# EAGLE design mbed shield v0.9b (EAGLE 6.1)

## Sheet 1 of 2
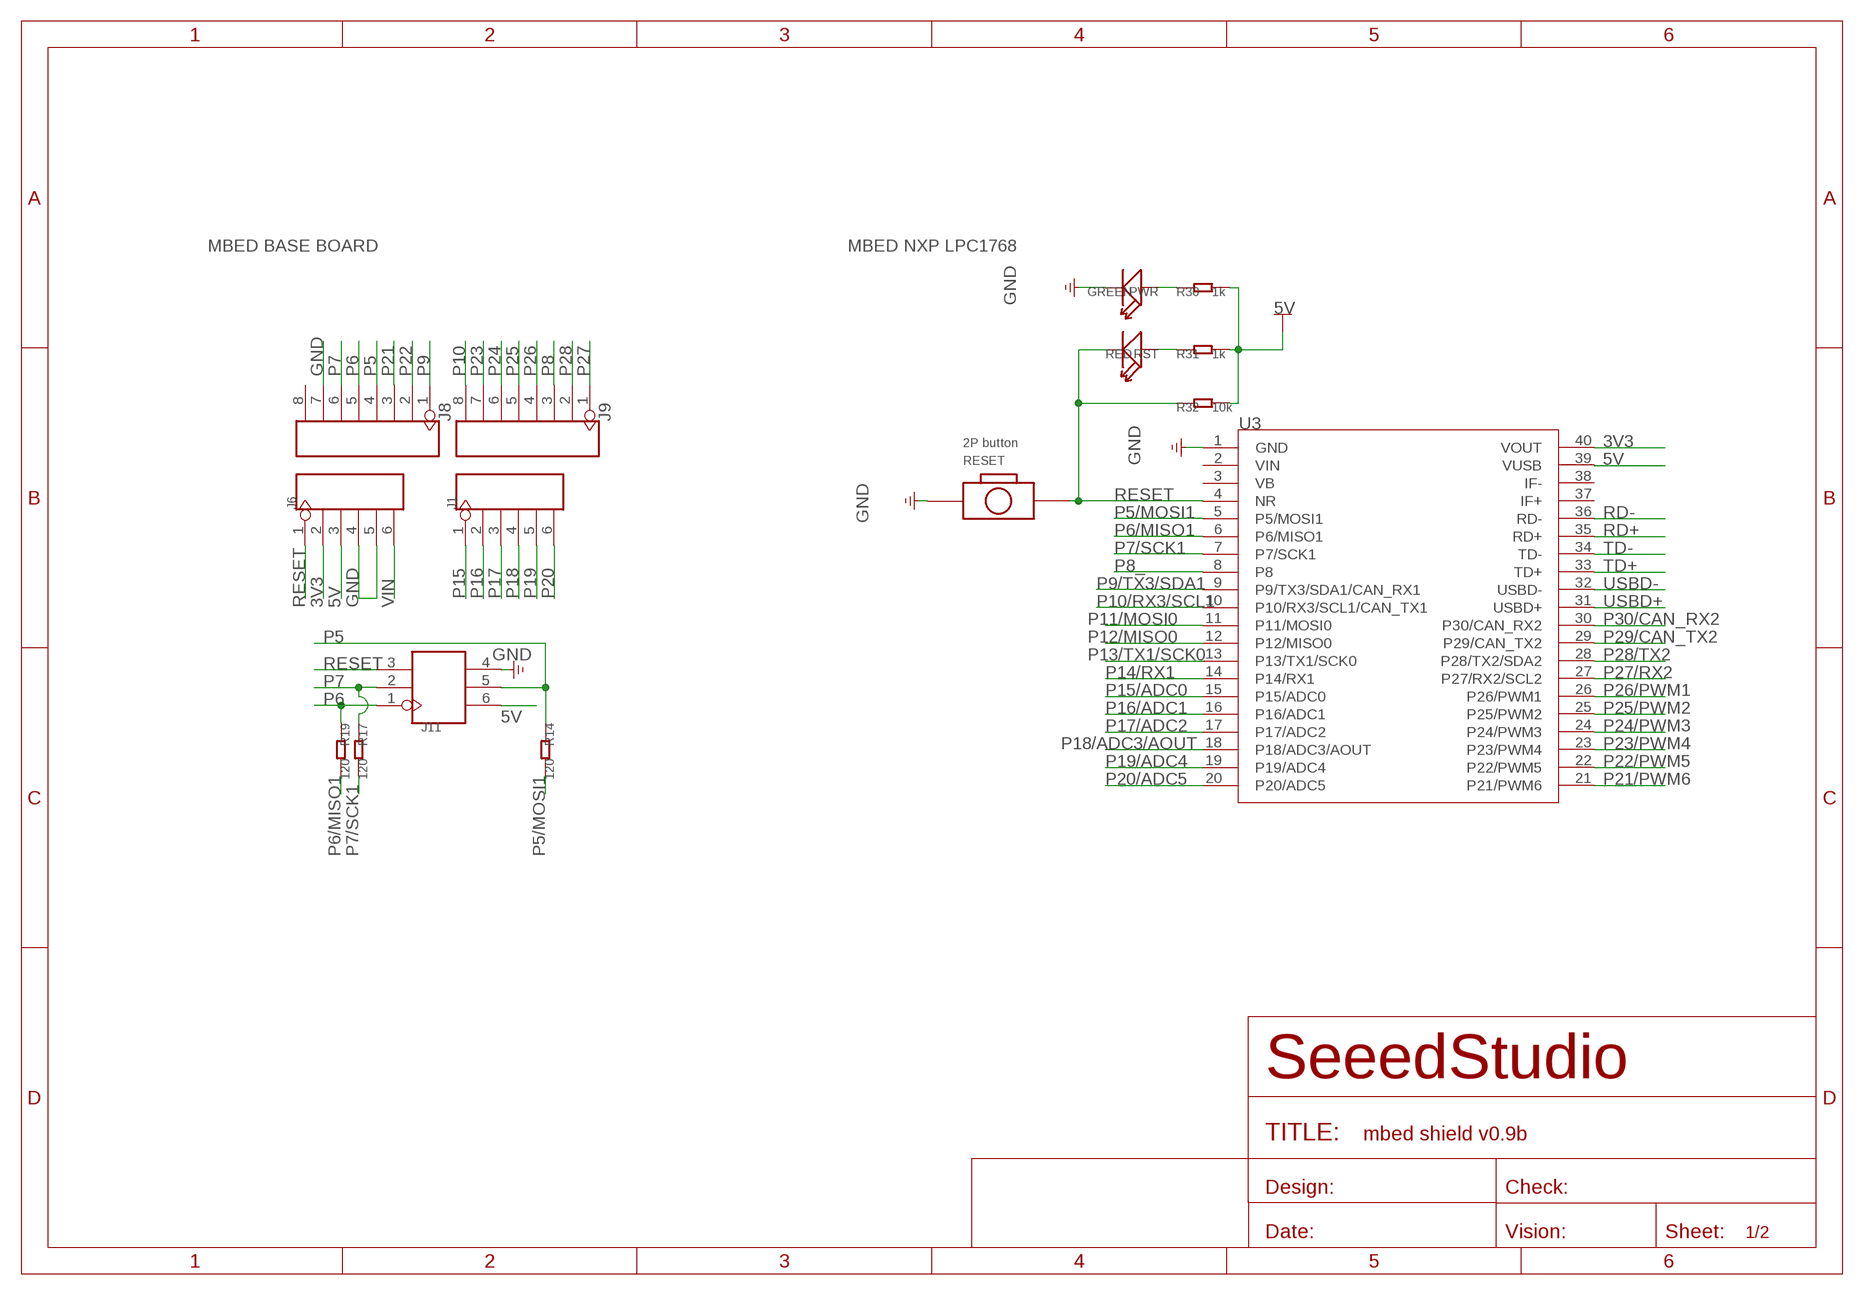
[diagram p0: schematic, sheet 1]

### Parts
J1  HEADER-6P-SMD  [6P-2.54-SMD]
J6  HEADER-6P-SMD  [6P-2.54-SMD]
J8  HEADER-8P-2.54-SMD  [8P-2.54-SMD]
J9  HEADER-8P-2.54-SMD  [8P-2.54-SMD]
J11  HEADER-2X3P-2.54  [2X3P-2.54]
PWR  GREEN  LED'0603'  [LED-0603]
R14  120  R-0603  [0603]
R17  120  R-0603  [0603]
R19  120  R-0603  [0603]
R30  1k  R-0603  [0603]
R31  1k  R-0603  [0603]
R32  10k  R-0603  [0603]
RESET  2P button  BOTTON-2P-90  [2P-7.62X3.56-90D]
RST  RED  LED'0603'  [LED-0603]
U3  MBED-LPC1768-SMD  [40P-SMD-2.54-53.34X36.67]

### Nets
3V3: J6.2 U3.40(VOUT) ; also sheet 2
5V: J6.3 J11.6 R30.2 R31.2 R32.2 U3.39(VUSB) ; also sheet 2
GND: J6.4 J6.5 J8.7 J11.4 PWR.- RESET.P$1 U3.1(GND) ; also sheet 2
N$2: R31.1 RST.+
N$3: PWR.+ R30.1
P5: J8.4 J11.5 R14.1
P5/MOSI1: R14.2 U3.5(P5/MOSI1)
P6: J8.5 J11.1 R19.1
P6/MISO1: R19.2 U3.6(P6/MISO1)
P7: J8.6 J11.2 R17.1
P7/SCK1: R17.2 U3.7(P7/SCK1)
P8: J9.3 ; also sheet 2
P8_: U3.8 ; also sheet 2
P9: J8.1 ; also sheet 2
P9/TX3/SDA1: U3.9(P9/TX3/SDA1/CAN_RX1) ; also sheet 2
P10: J9.8 ; also sheet 2
P10/RX3/SCL1: U3.10(P10/RX3/SCL1/CAN_TX1) ; also sheet 2
P11/MOSI0: U3.11(P11/MOSI0) ; also sheet 2
P12/MISO0: U3.12(P12/MISO0) ; also sheet 2
P13/TX1/SCK0: U3.13(P13/TX1/SCK0) ; also sheet 2
P14/RX1: U3.14(P14/RX1) ; also sheet 2
P15: J1.1 ; also sheet 2
P15/ADC0: U3.15(P15/ADC0) ; also sheet 2
P16: J1.2 ; also sheet 2
P16/ADC1: U3.16(P16/ADC1) ; also sheet 2
P17: J1.3 ; also sheet 2
P17/ADC2: U3.17(P17/ADC2) ; also sheet 2
P18: J1.4 ; also sheet 2
P18/ADC3/AOUT: U3.18(P18/ADC3/AOUT) ; also sheet 2
P19: J1.5 ; also sheet 2
P19/ADC4: U3.19(P19/ADC4) ; also sheet 2
P20: J1.6 ; also sheet 2
P20/ADC5: U3.20(P20/ADC5) ; also sheet 2
P21: J8.3 ; also sheet 2
P21/PWM6: U3.21(P21/PWM6) ; also sheet 2
P22: J8.2 ; also sheet 2
P22/PWM5: U3.22(P22/PWM5) ; also sheet 2
P23: J9.7 ; also sheet 2
P23/PWM4: U3.23(P23/PWM4) ; also sheet 2
P24: J9.6 ; also sheet 2
P24/PWM3: U3.24(P24/PWM3) ; also sheet 2
P25: J9.5 ; also sheet 2
P25/PWM2: U3.25(P25/PWM2) ; also sheet 2
P26: J9.4 ; also sheet 2
P26/PWM1: U3.26(P26/PWM1) ; also sheet 2
P27: J9.1 ; also sheet 2
P27/RX2: U3.27(P27/RX2/SCL2) ; also sheet 2
P28: J9.2 ; also sheet 2
P28/TX2: U3.28(P28/TX2/SDA2) ; also sheet 2
P29/CAN_TX2: U3.29(P29/CAN_TX2) ; also sheet 2
P30/CAN_RX2: U3.30(P30/CAN_RX2) ; also sheet 2
RD+: U3.35(RD+) ; also sheet 2
RD-: U3.36(RD-) ; also sheet 2
RESET: J6.1 J11.3 R32.1 RESET.P$2 RST.- U3.4(NR)
TD+: U3.33(TD+) ; also sheet 2
TD-: U3.34(TD-) ; also sheet 2
USBD+: U3.31(USBD+) ; also sheet 2
USBD-: U3.32(USBD-) ; also sheet 2
VIN: J6.6
Unconnected: J8.8 U3.2(VIN) U3.3(VB) U3.37(IF+) U3.38(IF-)

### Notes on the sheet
- MBED BASE BOARD | MBED NXP LPC1768

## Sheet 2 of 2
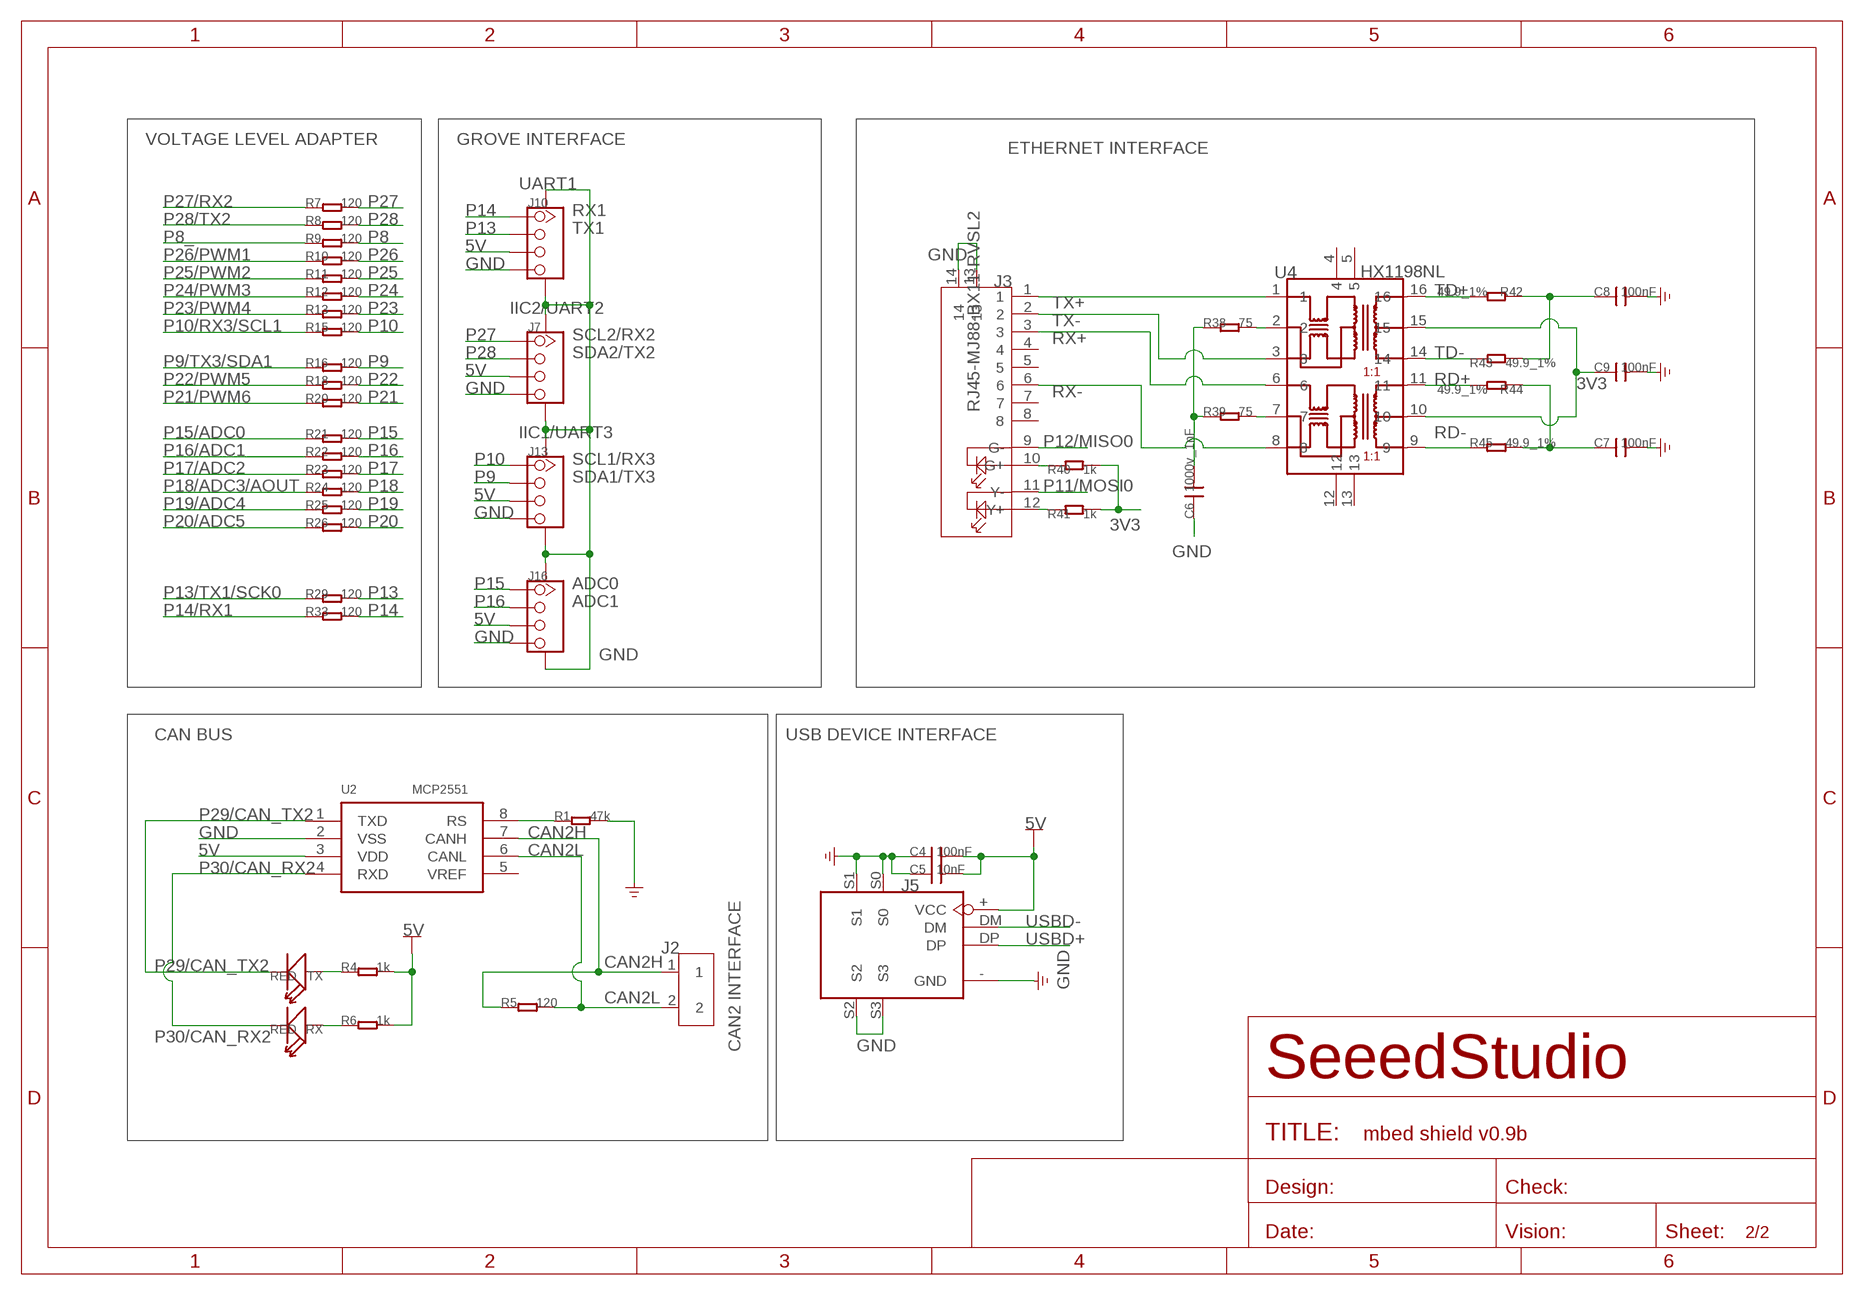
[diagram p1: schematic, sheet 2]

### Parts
C4  100nF  C-0603  [0603]
C5  10nF  C-0603  [0603]
C6  1000v_1nF  C  [C1206]
C7  100nF  C-0603  [0603]
C8  100nF  C-0603  [0603]
C9  100nF  C-0603  [0603]
J2  SCREW-TERMINAL-2P'3.5'  [2P-3.5]
J3  RJ45-MJ88-BX11-RVSL2  [RJ45-MJ88-BX11-RVSL2]
J5  USB-FEMALE-13.2X14.5  [FEMALE-14.5X13.2]
J7  TWIG-4P-2.0-SMD-FEMALE-REINFORCE'DD'  [4P-SMD-2.0]
J10  TWIG-4P-2.0-SMD-FEMALE-REINFORCE'DD'  [4P-SMD-2.0]
J13  TWIG-4P-2.0-SMD-FEMALE-REINFORCE'DD'  [4P-SMD-2.0]
J16  TWIG-4P-2.0-SMD-FEMALE-REINFORCE'DD'  [4P-SMD-2.0]
R1  47k  R-0603  [0603]
R4  1k  R-0603  [0603]
R5  120  R-0805  [0805]
R6  1k  R-0603  [0603]
R7  120  R-0603  [0603]
R8  120  R-0603  [0603]
R9  120  R-0603  [0603]
R10  120  R-0603  [0603]
R11  120  R-0603  [0603]
R12  120  R-0603  [0603]
R13  120  R-0603  [0603]
R15  120  R-0603  [0603]
R16  120  R-0603  [0603]
R18  120  R-0603  [0603]
R20  120  R-0603  [0603]
R21  120  R-0603  [0603]
R22  120  R-0603  [0603]
R23  120  R-0603  [0603]
R24  120  R-0603  [0603]
R25  120  R-0603  [0603]
R26  120  R-0603  [0603]
R29  120  R-0603  [0603]
R33  120  R-0603  [0603]
R38  75  R-0603  [0603]
R39  75  R-0603  [0603]
R40  1k  R-0603  [0603]
R41  1k  R-0603  [0603]
R42  49.9_1%  R-0603  [0603]
R43  49.9_1%  R-0603  [0603]
R44  49.9_1%  R-0603  [0603]
R45  49.9_1%  R-0603  [0603]
RX  RED  LED'0603'  [LED-0603]
TX  RED  LED'0603'  [LED-0603]
U2  MCP2551  [SO08]
U4  HX1198NL  [SOIC16-9.53]

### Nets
3V3: C9.1 R40.2 R41.2 U4.10 U4.15 ; also sheet 1
5V: C4.2 C5.2 J5.+(VCC) J7.3 J10.3 J13.3 J16.3 R4.2 R6.2 U2.3(VDD) ; also sheet 1
CAN2H: J2.1 R5.1 U2.7(CANH)
CAN2L: J2.2 R5.2 U2.6(CANL)
GND: C4.1 C5.1 C6.1 C7.2 C8.2 C9.2 J3.13 J3.14 J5.-(GND) J5.S0 J5.S1 J5.S2 J5.S3 J7.4 J7.SS1 J7.SS2 J10.4 J10.SS1 J10.SS2 J13.4 J13.SS1 J13.SS2 J16.4 J16.SS1 J16.SS2 R1.2 U2.2(VSS) ; also sheet 1
N$1: R39.2 U4.7
N$4: R38.2 U4.2
N$5: C6.2 R38.1 R39.1
N$6: C7.1 R44.1 R45.2
N$7: C8.1 R42.1 R43.2
N$11: J3.12(Y+) R41.1
N$12: J3.10(G+) R40.1
N$20: R1.1 U2.8(RS)
N$46: R4.1 TX.+
N$47: R6.1 RX.+
P8: R9.2 ; also sheet 1
P8_: R9.1 ; also sheet 1
P9: J13.2 R16.2 ; also sheet 1
P9/TX3/SDA1: R16.1 ; also sheet 1
P10: J13.1 R15.2 ; also sheet 1
P10/RX3/SCL1: R15.1 ; also sheet 1
P11/MOSI0: J3.11(Y-) ; also sheet 1
P12/MISO0: J3.9(G-) ; also sheet 1
P13: J10.2 R29.2
P13/TX1/SCK0: R29.1 ; also sheet 1
P14: J10.1 R33.2
P14/RX1: R33.1 ; also sheet 1
P15: J16.1 R21.2 ; also sheet 1
P15/ADC0: R21.1 ; also sheet 1
P16: J16.2 R22.2 ; also sheet 1
P16/ADC1: R22.1 ; also sheet 1
P17: R23.2 ; also sheet 1
P17/ADC2: R23.1 ; also sheet 1
P18: R24.2 ; also sheet 1
P18/ADC3/AOUT: R24.1 ; also sheet 1
P19: R25.2 ; also sheet 1
P19/ADC4: R25.1 ; also sheet 1
P20: R26.2 ; also sheet 1
P20/ADC5: R26.1 ; also sheet 1
P21: R20.2 ; also sheet 1
P21/PWM6: R20.1 ; also sheet 1
P22: R18.2 ; also sheet 1
P22/PWM5: R18.1 ; also sheet 1
P23: R13.2 ; also sheet 1
P23/PWM4: R13.1 ; also sheet 1
P24: R12.2 ; also sheet 1
P24/PWM3: R12.1 ; also sheet 1
P25: R11.2 ; also sheet 1
P25/PWM2: R11.1 ; also sheet 1
P26: R10.2 ; also sheet 1
P26/PWM1: R10.1 ; also sheet 1
P27: J7.1 R7.2 ; also sheet 1
P27/RX2: R7.1 ; also sheet 1
P28: J7.2 R8.2 ; also sheet 1
P28/TX2: R8.1 ; also sheet 1
P29/CAN_TX2: TX.- U2.1(TXD) ; also sheet 1
P30/CAN_RX2: RX.- U2.4(RXD) ; also sheet 1
RD+: R44.2 U4.11 ; also sheet 1
RD-: R45.1 U4.9 ; also sheet 1
RX+: J3.3 U4.6
RX-: J3.6 U4.8
TD+: R42.2 U4.16 ; also sheet 1
TD-: R43.1 U4.14 ; also sheet 1
TX+: J3.1 U4.1
TX-: J3.2 U4.3
USBD+: J5.DP ; also sheet 1
USBD-: J5.DM ; also sheet 1
Unconnected: J3.4 J3.5 J3.7 J3.8 U2.5(VREF) U4.4 U4.5 U4.12 U4.13

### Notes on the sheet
- VOLTAGE LEVEL ADAPTER | GROVE INTERFACE
- ETHERNET INTERFACE
- UART1
- RX1
- TX1
- IIC2/UART2
- SCL2/RX2
- SDA2/TX2
- IIC1/UART3
- SCL1/RX3
- SDA1/TX3
- ADC0
- ADC1
- CAN BUS | USB DEVICE INTERFACE
- CAN2 INTERFACE

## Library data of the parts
C4-C9 = Discrete:C*: Ceramic Capacitors
J1 J6 = Connector:HEADER-6P
J2 = Connector:SCREW-TERMINAL-2P
J3 = Connector:RJ45-MJ88-BX11-RVSL2: Modular Jack 8P8C,R/A,With LED
J5 = Connector:USB-FEMALE
J7 J10 J13 J16 = Connector:TWIG-4P-2.0-SMD-FEMALE-REINFORCE
J8 J9 = Connector:HEADER-8P
J11 = Connector:HEADER-2X3P
PWR RST RX TX = Discrete:LED*
R1 R4-R26 R29-R33 R38-R45 = Discrete:R*
RESET = Discrete:BOTTON-2P
U2 = IC:MCP2551
U3 = template:MBED-LPC1768: MBED NXP LC1768外形及其对应排母
U4 = IC:HX1198NL: 10/100BASE-T Single Port Surface Mount Magnetics With Various Turns Ratios

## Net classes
0 default: width 0.203 mm, drill 0.305 mm, clearance 0.152 mm
3 usbvcc: width 0.203 mm, drill 0.305 mm, clearance 0.203 mm

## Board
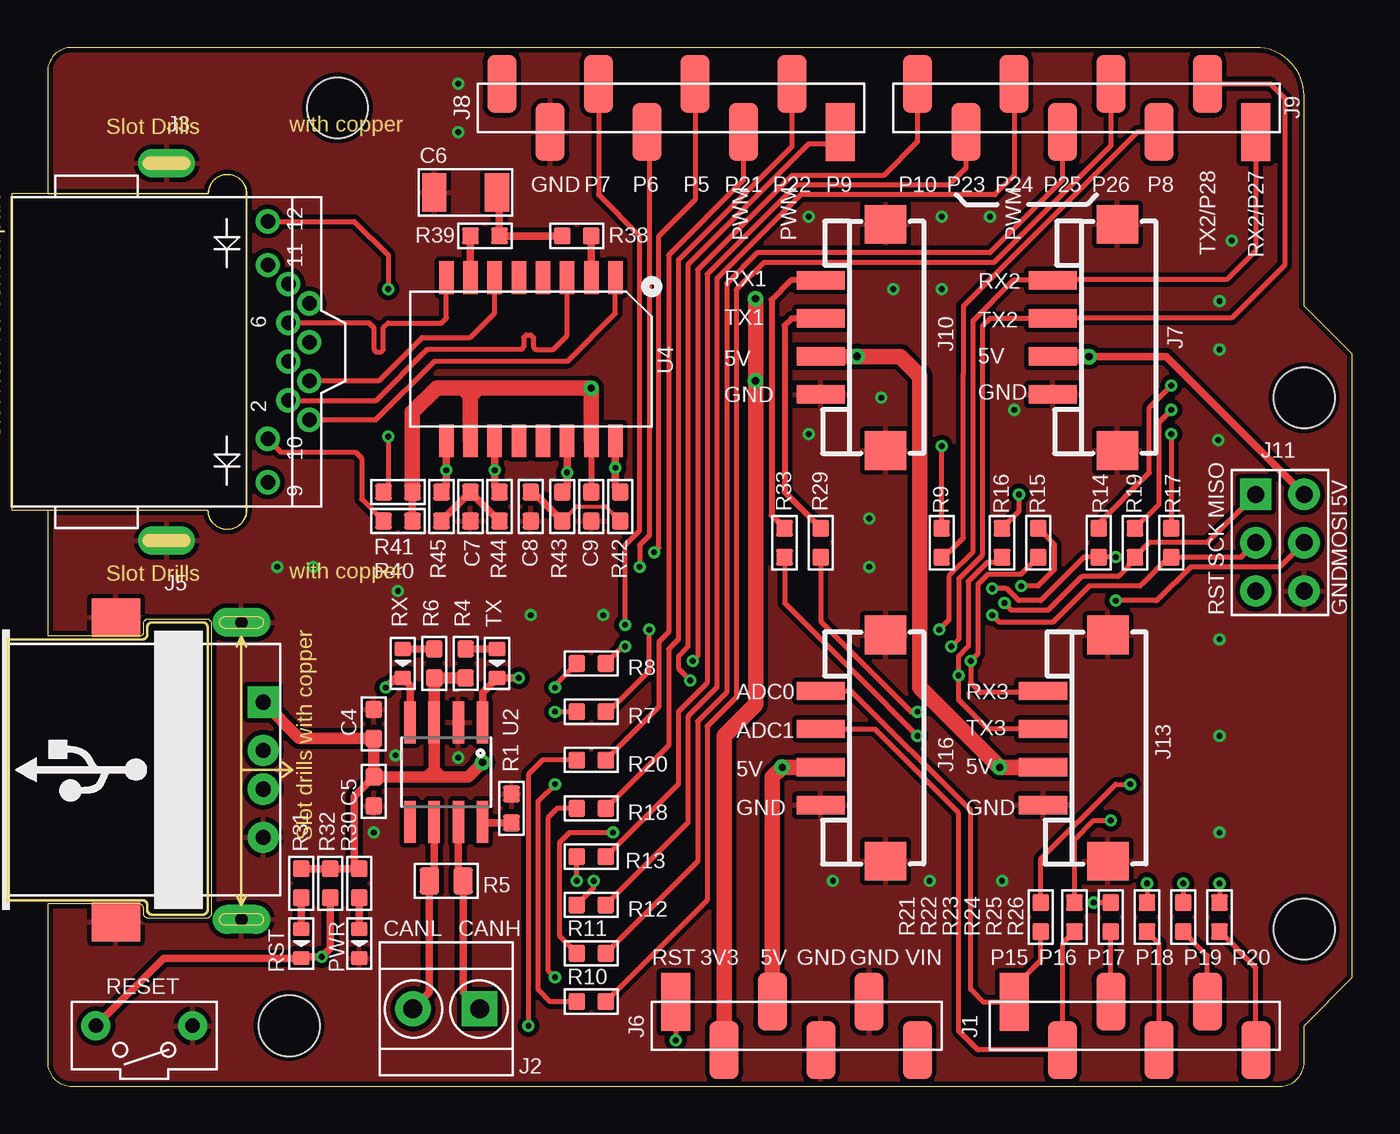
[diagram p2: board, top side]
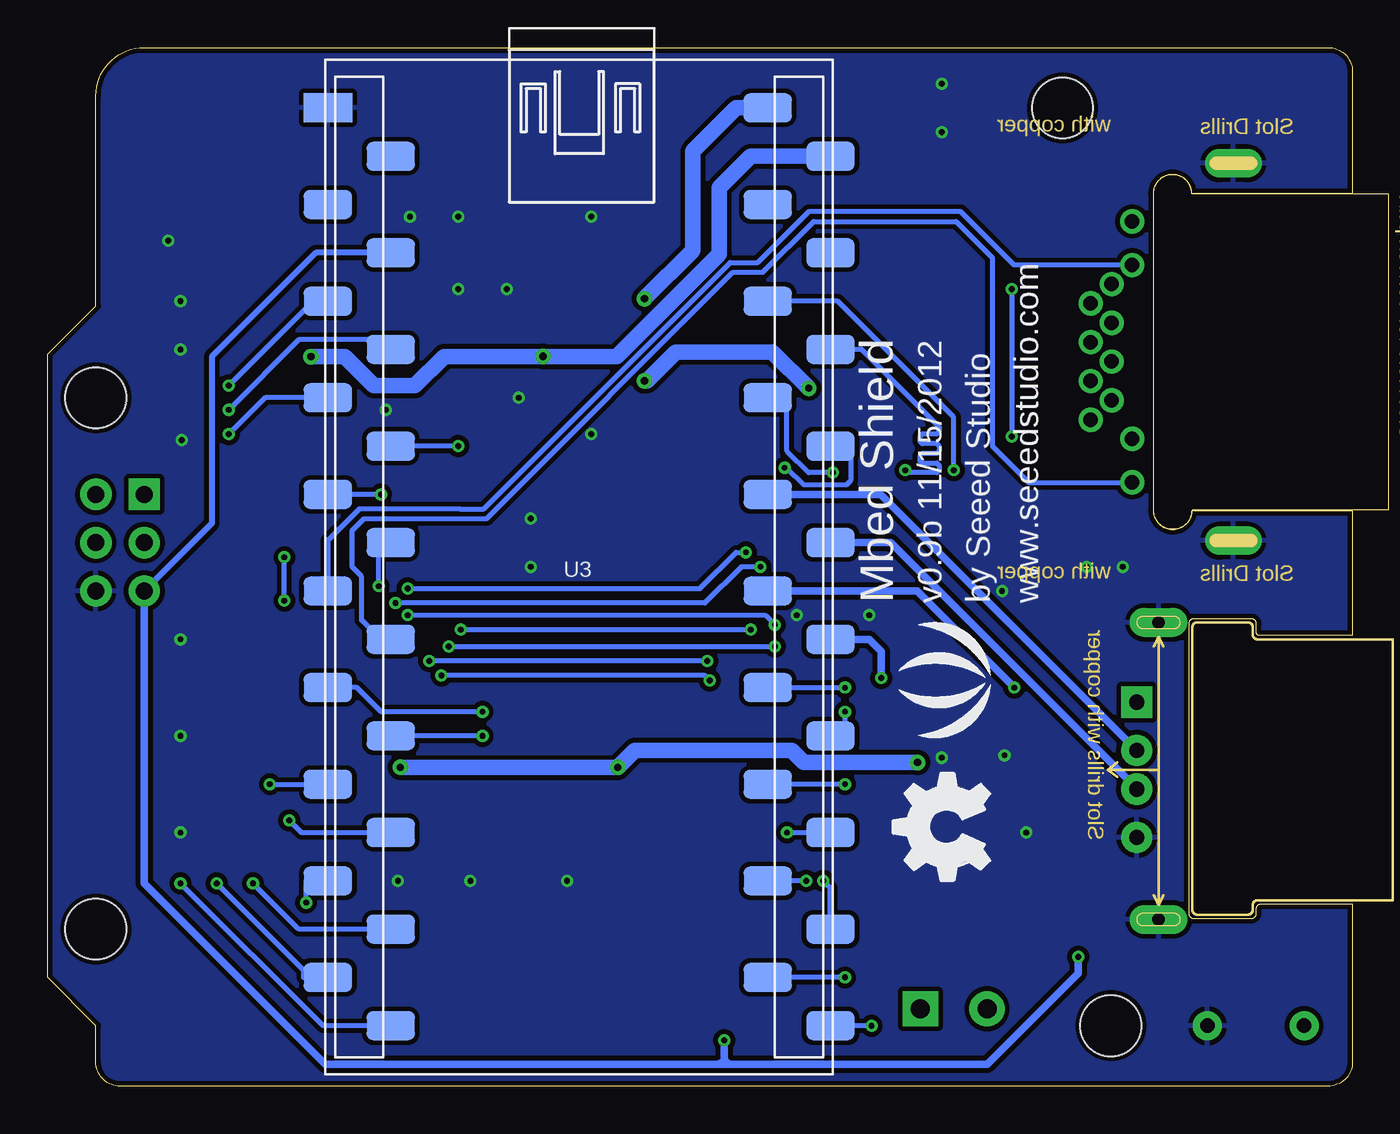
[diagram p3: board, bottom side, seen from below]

Size 68.58 x 54.61 mm. Coordinates in mm from the lower left corner, seen from the top.
Outline: 66.04,41.02 66.04,52.07 arc90 63.5,54.61 1.27,54.61 arc90 0,53.34 0,46.94 8.45,46.94 arc-90 9.45,47.94 9.46,47.94 arc-90 10.47,46.92 10.47,30.29 arc-90 9.46,29.27 9.43,29.27 arc-90 8.43,30.28 0,30.28 0,23.7 4.9,23.7 arc90 5.05,23.85 5.05,24.32 arc-90 5.3,24.57 8.35,24.57 arc-90 8.6,24.32 8.6,9.08 arc-90 8.35,8.83 5.3,8.83 arc-90 5.05,9.08 5.05,9.33 arc90 4.79,9.59 0,9.59 0,1.27 arc90 1.27,0 64.77,0 arc90 66.04,1.27 66.04,3.17 68.58,5.71 68.58,38.48 66.04,41.02
Copper layers (1*16): Top 0.035mm / dielectric 1.5mm / Bottom 0.035mm
Design rules: minimum track width 6mil, minimum drill 12mil, track to track 6mil, track to pad 6mil, pad to pad 6mil, via to via 6mil, smd to smd 0mil, copper to edge 10mil, drill to drill 10mil, minimum pad ring 10mil, minimum via ring 6mil, stop-mask expansion 2mil, vias tented up to drill 100mil, thermal gap 10mil
Holes 3.2 mm at 15.24,51.43 66.04,36.2 66.04,8.26 12.7,3.17

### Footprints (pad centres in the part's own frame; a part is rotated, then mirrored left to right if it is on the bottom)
0603 = smd 0.889 x 0.889: 1 -0.762,0; 2 0.762,0
C1206 = smd 1.27 x 2.032: 1 -1.651,0; 2 1.651,0
6P-2.54-SMD = smd 3.048 x 1.524: 1 1.27,6.35; 2 -1.27,3.81; 3 1.27,1.27; 4 -1.27,-1.27; 5 1.27,-3.81; 6 -1.27,-6.35
2P-3.5 = drill 1 pad 1.85 square: 1 -1.75,0 | drill 1 pad 1.85: 2 1.75,0
RJ45-MJ88-BX11-RVSL2 = drill 0.762 pad 1.27: 1 3.57,7.5; 2 2.55,6.4; 3 1.53,7.5; 4 0.51,6.4; 5 -0.51,7.5; 6 -1.53,6.4; 7 -2.55,7.5; 8 -3.57,6.4; 9 6.86,5.32; 10 4.57,5.32; 11 -4.57,5.32; 12 -6.86,5.32 | drill 0.6 pad 1.5 long: 13 -9.92,0; 14 9.92,0
FEMALE-14.5X13.2 = drill 0.813 pad 1.651 square: + 0.889,-3.556 | drill 0.813 pad 1.651: - 0.889,3.556; DM 0.889,-1.016; DP 0.889,1.016 | smd 2.54 x 2.032: S0 8.636,8.001; S3 8.636,-8.001 | drill 0.635 pad 1.524 long: S1 2.032,7.874; S2 2.032,-7.747
4P-SMD-2.0 = smd 0.965 x 2.54: 1 -3,0; 2 -1,0; 3 1,0; 4 3,0 | smd 2.032 x 2.184: SS1 -5.946,3.4; SS2 5.946,3.4
8P-2.54-SMD = smd 3.048 x 1.524: 1 1.27,8.89; 2 -1.27,6.35; 3 1.27,3.81; 4 -1.27,1.27; 5 1.27,-1.27; 6 -1.27,-3.81; 7 1.27,-6.35; 8 -1.27,-8.89
2X3P-2.54 = drill 0.889 pad 1.651 square: 1 -1.27,2.54 | drill 0.889 pad 1.651: 2 -1.27,0; 3 -1.27,-2.54; 4 1.27,-2.54; 5 1.27,0; 6 1.27,2.54
LED-0603 = smd 0.762 x 0.889: + -0.762,0; - 0.762,0
0805 = smd 1.016 x 1.397: 1 -0.889,0; 2 0.889,0
2P-7.62X3.56-90D = drill 0.762 pad 1.524: P$1 0,2.54; P$2 0,-2.54
SO08 = smd 0.61 x 2.21: 1 -1.905,-2.616; 2 -0.635,-2.616; 3 0.635,-2.616; 4 1.905,-2.616; 5 1.905,2.616; 6 0.635,2.616; 7 -0.635,2.616; 8 -1.905,2.616
40P-SMD-2.54-53.34X36.67 = smd 1.524 x 2.54: 1 -24.13,-13.208; 2 -21.59,-9.906; 3 -19.05,-13.208; 4 -16.51,-9.906; 5 -13.97,-13.208; 6 -11.43,-9.906; 7 -8.89,-13.208; 8 -6.35,-9.906; 9 -3.81,-13.208; 10 -1.27,-9.906; 11 1.27,-13.208; 12 3.81,-9.906; 13 6.35,-13.208; 14 8.89,-9.906; 15 11.43,-13.208; 16 13.97,-9.906; 17 16.51,-13.208; 18 19.05,-9.906; 19 21.59,-13.208; 20 24.13,-9.906; 21 24.13,13.208; 22 21.59,9.906; 23 19.05,13.208; 24 16.51,9.906; 25 13.97,13.208; 26 11.43,9.906; 27 8.89,13.208; 28 6.35,9.906; 29 3.81,13.208; 30 1.27,9.906; 31 -1.27,13.208; 32 -3.81,9.906; 33 -6.35,13.208; 34 -8.89,9.906; 35 -11.43,13.208; 36 -13.97,9.906; 37 -16.51,13.208; 38 -19.05,9.906; 39 -21.59,13.208; 40 -24.13,9.906
SOIC16-9.53 = smd 0.762 x 1.714: 1 -4.445,-4.286; 2 -3.175,-4.286; 3 -1.905,-4.286; 4 -0.635,-4.286; 5 0.635,-4.286; 6 1.905,-4.286; 7 3.175,-4.286; 8 4.445,-4.286; 9 4.445,4.286; 10 3.175,4.286; 11 1.905,4.286; 12 0.635,4.286; 13 -0.635,4.286; 14 -1.905,4.286; 15 -3.175,4.286; 16 -4.445,4.286

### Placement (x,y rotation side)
C4  17.14,19.05 270 top
C5  17.14,15.49 90 top
C6  21.97,46.99 0 top
C7  22.23,30.48 270 top
C8  25.4,30.48 270 top
C9  28.57,30.48 270 top
J1  57.15,3.17 90 top
J2  20.95,4.06 180 top
J3  6.25,38.61 270 top
J5  12.22,16.64 180 top
J6  39.37,3.17 90 top
J7  52.83,39.37 270 top
J8  32.77,51.43 270 top
J9  54.61,51.43 270 top
J10  40.64,39.37 270 top
J11  64.77,28.58 0 top
J13  52.32,17.78 270 top
J16  40.64,17.78 270 top
PWR  16.38,7.49 270 top
R1  24.38,14.61 90 top
R4  21.97,22.23 270 top
R5  20.95,10.79 180 top
R6  20.32,22.23 270 top
R7  28.57,19.69 0 top
R8  28.57,22.23 0 top
R9  46.99,28.58 270 top
R10  28.57,4.45 0 top
R11  28.57,6.98 0 top
R12  28.57,9.53 0 top
R13  28.57,12.06 0 top
R14  55.24,28.58 90 top
R15  52.07,28.58 270 top
R16  50.16,28.58 270 top
R17  59.05,28.58 90 top
R18  28.57,14.61 0 top
R19  57.15,28.58 90 top
R20  28.57,17.15 0 top
R21  52.2,8.89 270 top
R22  53.98,8.89 270 top
R23  55.88,8.89 270 top
R24  57.78,8.89 270 top
R25  59.69,8.89 270 top
R26  61.59,8.89 270 top
R29  40.64,28.58 90 top
R30  16.38,10.67 90 top
R31  13.34,10.67 90 top
R32  14.86,10.67 90 top
R33  38.73,28.58 90 top
R38  27.81,44.7 0 top
R39  22.99,44.7 180 top
R40  18.41,29.72 0 top
R41  18.41,31.24 0 top
R42  30.1,30.48 90 top
R43  27.05,30.48 270 top
R44  23.75,30.48 90 top
R45  20.7,30.48 270 top
RESET  5.08,3.17 270 top
RST  13.34,7.49 270 top
RX  18.67,22.23 270 top
TX  23.62,22.23 270 top
U2  20.95,16.51 180 top
U3  40.64,27.31 270 bottom
U4  25.4,38.23 180 top
U$15  [LOGO_SILK]  20.7,21.34 90 bottom
U$16  [OSHW_FILLX200_NOTEXT]  19.05,10.79 90 bottom

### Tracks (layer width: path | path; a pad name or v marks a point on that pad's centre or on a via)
3V3  (via drill 0.38 pad 0.81)
  Top 0.305: U4.15 C9.1
  Top 0.406: R40.2 R41.2
  Top 0.813: J6.2 35.56,18.42 37.21,20.07 v37.21,37.08 v37.21,41.4 | U4.15 v28.57,36.7 22.61,36.7 | R41.2 19.18,35.43 20.45,36.7 21.84,36.7 | 21.84,36.7 22.48,36.7 | 22.48,36.7 22.61,36.7 | U4.10 22.23,36.32 | 22.23,36.32 22.23,36.45 22.48,36.7 | 22.23,36.32 21.84,36.7 | 22.23,36.32 22.61,36.7
  Bottom 0.813: v37.21,37.08 37.08,37.08 35.56,38.61 30.48,38.61 v28.57,36.7 | U3.40 32.38,51.43 34.67,49.15 34.67,43.94 v37.21,41.4
5V  (via drill 0.38 pad 0.81)
  Top 0.406: R31.2 R32.2 16.13,11.43 | R30.2 16.13,11.43 | 16.13,11.43 16.13,15.24 C5.2 | v54.74,38.35 58.8,38.35 J11.6
  Top 0.61: R4.2 R6.2 U2.3 20.32,16.64 | J5.+ 13.24,18.29 C4.2 C5.2 19.94,16.26 | 19.94,16.26 20.32,16.64 | 19.94,16.26 20.7,16.26 | 20.7,16.26 22.1,16.26 v22.86,17.02 | 20.32,16.64 20.7,16.26
  Top 0.813: J6.3 38.1,16.26 v38.61,16.76 40.62,16.76 J16.3 | J10.3 v42.55,38.37 44.81,38.37 45.85,37.34 45.85,20.96 v50.04,16.76 52.31,16.76 J13.3 | v54.74,38.35 52.85,38.35 J7.3
  Bottom 0.813: U3.39 31.62,48.89 33.27,47.24 33.27,43.75 38.66,38.37 v42.55,38.37 47.74,38.37 49.28,36.83 51.44,36.83 52.96,38.35 v54.74,38.35 | v22.86,17.02 28.83,17.02 29.46,17.65 37.72,17.65 v38.61,16.76 v50.04,16.76
CAN2H
  Top 0.406: U2.7 21.59,11.05 R5.1 21.84,4.92 J2.1
CAN2L
  Top 0.406: U2.6 20.32,11.05 R5.2 20.07,4.92 J2.2
GND  (via drill 0.3 pad 0.64)
  other vias: 25.4,24.77 12.06,27.31 13.97,27.31 18.41,26.04 40.01,34.29 43.18,27.31 43.81,36.2 46.99,45.72 49.53,45.72 62.23,44.45 61.59,41.27 61.59,38.73 29.21,24.77 41.27,10.79 46.35,10.79 50.16,10.79 61.59,23.5 61.59,18.42 61.59,13.33 17.14,13.33 21.59,17.27 18.29,17.4 43.18,29.85 50.8,35.56 40.01,45.72 46.99,41.91 44.45,41.91 61.53,33.97 21.59,52.7 21.59,50.16
  pour Top: -9.53,52.7 -8.38,52.7 -8.26,52.58 -8.26,51.43 -9.4,51.43 -9.53,51.56
  pour Top (isolate 0.254): 0,54.61 68.58,54.61 68.58,0 0,0
  pour Bottom (isolate 0.254): 0,54.61 68.58,54.61 68.58,0 0,0
N$1
  Top 0.406: U4.7 R39.2
N$2
  Top 0.406: R31.1 RST.+
N$3
  Top 0.406: R30.1 PWR.+
N$4
  Top 0.406: U4.2 R38.2
N$5
  Top 0.406: R38.1 R39.1 23.75,46.86 C6.2
N$6
  Top 0.406: R45.2 21.46,30.48 C7.1 23.11,30.35 R44.1
N$7
  Top 0.203: R43.2 27.81,30.48 29.34,30.48 R42.1
  Top 0.406: C8.1 25.53,31.24 26.29,30.48 R43.2
N$11  (via drill 0.3 pad 0.64)
  Top 0.254: J3.12 16.13,45.47 17.91,43.69 v17.91,41.91 | v17.91,34.16 17.91,31.5 R41.1
  Bottom 0.254: v17.91,41.91 v17.91,34.16
N$12
  Top 0.254: J3.10 11.57,34.02 12.26,33.34 16.19,33.34 16.51,33.02 16.51,30.86 R40.1
N$20
  Top 0.406: R1.1 22.91,13.84 U2.8
N$46
  Top 0.406: R4.1 TX.+
N$47
  Top 0.406: RX.+ R6.1
P5  (via drill 0.3 pad 0.64)
  Top 0.254: R14.1 55.24,27.69 | J8.4 34.04,46.61 32.13,44.7 32.13,28.32 v31.88,28.07 | R14.1 54.48,27.81 52.2,25.53 51.05,25.53 50.42,26.16 v49.66,26.16 | J11.5 64.77,27.31 60.07,27.31 58.29,25.53 v56.13,25.53 | v56.13,27.81 R14.1
  Bottom 0.254: v49.66,26.16 34.29,26.16 32.38,28.07 v31.88,28.07 | v56.13,25.53 v56.13,27.81
P5/MOSI1  (via drill 0.3 pad 0.64)
  Top 0.254: R14.2 55.24,29.59 57.91,32.26 57.91,35.69 v59.05,36.83
  Bottom 0.254: U3.5 54.61,41.27 v59.05,36.83
P6  (via drill 0.3 pad 0.64)
  Top 0.254: J8.5 31.5,49.78 31.62,49.66 31.62,28.96 31.11,28.45 v31.11,27.31 | v50.29,25.4 50.67,25.02 52.58,25.02 54.36,26.8 56.26,26.8 57.15,27.69 R19.1 57.91,28.58 60.96,28.58 J11.1
  Bottom 0.254: v31.11,27.31 32.13,27.31 34.04,25.4 v50.29,25.4
P6/MISO1  (via drill 0.3 pad 0.64)
  Top 0.254: R19.2 58.42,30.61 58.42,34.92 v59.05,35.56
  Bottom 0.254: 49.78,38.48 50.04,38.73 U3.6 50.67,38.73 51.18,39.24 55.37,39.24 v59.05,35.56
P7  (via drill 0.3 pad 0.64)
  Top 0.254: J8.6 28.96,46.86 31.11,44.7 31.11,29.21 30.35,28.45 v30.35,24.26 | J11.2 62.74,27.81 R17.1 58.93,27.81 57.53,26.42 57.4,26.29 54.74,26.29 52.83,24.38 50.04,24.38 v49.66,24.77
  Bottom 0.254: v49.66,24.77 30.86,24.77 v30.35,24.26
P7/SCK1  (via drill 0.3 pad 0.64)
  Top 0.254: v59.05,34.29 R17.2
  Bottom 0.254: U3.7 57.15,36.2 v59.05,34.29
P8
  Top 0.254: J9.3 57.28,50.16 48.13,41.02 48.13,37.46 48.13,28.83 47.12,27.81 R9.2
P8_  (via drill 0.3 pad 0.64)
  Top 0.254: R9.1 v46.99,33.66
  Bottom 0.254: 51.18,33.66 U3.8 v46.99,33.66
P9  (via drill 0.3 pad 0.64)
  Top 0.254: J8.1 41.66,49.53 39.98,49.53 33.66,43.2 33.66,23.11 33.15,22.61 33.15,21.97 v33.78,21.34 | 52.31,18.8 J13.2 49.42,18.78 47.88,20.32 v47.88,21.59 47.88,22.61 48.39,23.11 48.39,26.54 49.4,27.56 49.91,27.56 R16.2
  Bottom 0.254: v33.78,21.34 34.04,21.59 v47.88,21.59
P9/TX3/SDA1  (via drill 0.3 pad 0.64)
  Top 0.254: v51.05,31.12 51.05,30.23 R16.1
  Bottom 0.254: v51.05,31.12 U3.9
P10  (via drill 0.3 pad 0.64)
  Top 0.254: J9.8 45.72,49.66 43.94,47.88 39.1,47.88 34.16,42.94 34.16,22.61 v33.91,22.35 | J13.1 52.24,20.7 49.02,20.7 48.51,21.21 v48.51,22.35 48.9,22.73 48.9,26.39 49.43,26.92 51.18,26.92 R15.2
  Bottom 0.254: v33.91,22.35 v48.51,22.35
P10/RX3/SCL1  (via drill 0.3 pad 0.64)
  Top 0.254: R15.1 52.92,28.49 52.92,27.16 52.05,26.29 v51.18,26.29
  Bottom 0.254: v51.18,26.29 51.18,27.94 U3.10
P11/MOSI0
  Bottom 0.254: J3.11 17.78,43.18 20.57,45.97 28.57,45.97 31.24,43.31 32.7,43.31 45.66,30.35 46.93,30.35 52.2,30.35 53.85,28.7 U3.11
P12/MISO0
  Bottom 0.254: J3.9 17.02,31.75 18.92,33.66 18.92,43.56 20.83,45.47 28.32,45.47 30.99,42.8 32.56,42.8 45.51,29.85 51.94,29.85 52.58,29.21 52.58,27.31 52.07,26.8 52.07,24.51 51.05,23.5 U3.12
P13
  Top 0.305: R29.2 38.73,31.24 38.73,40 39.1,40.37 J10.2
P13/TX1/SCK0  (via drill 0.3 pad 0.64)
  Top 0.254: R29.1 40.64,24.43 45.39,19.69 v45.72,19.69
  Bottom 0.254: v45.72,19.69 51.05,19.69 52.32,20.96 U3.13
P14
  Top 0.305: J10.1 39.07,42.37 38.05,41.35 38.05,30.02 R33.2
P14/RX1  (via drill 0.3 pad 0.64)
  Top 0.254: R33.1 38.73,25.4 42.55,21.59 v45.72,18.42
  Bottom 0.254: 51.18,18.42 U3.14 v45.72,18.42
P15
  Top 0.254: J16.1 42.23,20.78 48.51,14.49 48.51,5.08 49.15,4.45 J1.1 50.8,5.21 52.2,6.6 R21.2
P15/ADC0  (via drill 0.3 pad 0.64)
  Top 0.254: v56.9,15.88 56.13,15.88 52.2,11.94 R21.1
  Bottom 0.254: v56.9,15.88 U3.15
P16
  Top 0.254: J16.2 43.47,18.78 47.88,14.37 47.88,2.92 48.9,1.91 J1.2 53.34,7.49 R22.2
P16/ADC1  (via drill 0.3 pad 0.64)
  Top 0.254: v55.88,13.97 54.99,13.97 53.98,12.95 R22.1
  Bottom 0.254: v55.88,13.97 55.24,13.33 U3.16
P17
  Top 0.254: J1.3 R23.2
P17/ADC2  (via drill 0.3 pad 0.64)
  Top 0.254: v54.99,9.65 R23.1
  Bottom 0.254: 53.98,10.79 U3.17 54.99,10.79 v54.99,9.65
P18
  Top 0.254: J1.4 58.42,7.49 R24.2
P18/ADC3/AOUT  (via drill 0.3 pad 0.64)
  Top 0.254: v57.78,10.67 R24.1
  Bottom 0.254: U3.18 55.37,8.26 v57.78,10.67
P19
  Top 0.254: J1.5 60.96,6.86 R25.2
P19/ADC4  (via drill 0.3 pad 0.64)
  Top 0.254: v59.69,10.67 R25.1
  Bottom 0.254: U3.19 55.12,5.71 55.12,6.1 v59.69,10.67
P20
  Top 0.254: 61.59,8 R26.2 63.5,6.22 J1.6
P20/ADC5  (via drill 0.3 pad 0.64)
  Top 0.254: v61.59,10.67 R26.1
  Bottom 0.254: v61.59,10.67 54.1,3.17 U3.20
P21
  Top 0.254: R20.2 32.13,19.94 32.13,23.37 32.64,23.88 32.64,43.69 36.58,47.62 J8.3
P21/PWM6  (via drill 0.3 pad 0.64)
  Top 0.254: R20.1 26.04,17.15 25.27,16.38 v25.27,3.17
  Bottom 0.254: v25.27,3.17 U3.21
P22
  Top 0.254: R18.2 32.64,17.91 32.64,22.99 33.15,23.5 33.15,43.43 39.12,49.4 J8.2
P22/PWM5  (via drill 0.3 pad 0.64)
  Top 0.254: R18.1 26.8,14.61 26.29,14.1 26.29,6.1 v26.67,5.71
  Bottom 0.254: v26.67,5.71 U3.22
P23
  Top 0.254: J9.7 48.26,48.26 47.37,47.37 39.34,47.37 34.67,42.7 34.67,21.21 33.15,19.69 33.15,15.88 R13.2
P23/PWM4  (via drill 0.3 pad 0.64)
  Top 0.254: v27.81,10.79 R13.1
  Bottom 0.254: U3.23 27.43,10.41 v27.81,10.79
P24
  Top 0.254: J9.6 50.8,47.88 49.78,46.86 39.58,46.86 35.18,42.46 35.18,20.96 33.66,19.43 33.66,13.84 R12.2
P24/PWM3  (via drill 0.3 pad 0.64)
  Top 0.254: R12.1 28.7,10.41 v28.7,10.79
  Bottom 0.254: v28.7,10.79 U3.24
P25
  Top 0.254: J9.5 53.34,47.62 49.53,43.81 37.3,43.81 35.69,42.2 35.69,20.7 34.16,19.18 34.16,11.81 R11.2
P25/PWM2  (via drill 0.3 pad 0.64)
  Top 0.254: R11.1 26.92,7.87 26.92,12.83 U3.25 v29.72,13.33
  Bottom 0.254: v29.72,13.33 U3.25
P26
  Top 0.254: J9.4 55.88,49.45 49.73,43.31 37.63,43.31 36.2,41.87 36.2,20.45 34.67,18.92 34.67,9.78 R10.2
P26/PWM1  (via drill 0.3 pad 0.64)
  Top 0.254: R10.1 26.42,4.45 25.78,5.08 25.78,14.99 v26.67,15.88
  Bottom 0.254: v26.67,15.88 U3.26
P27  (via drill 0.3 pad 0.64)
  Top 0.254: 52.82,42.35 J7.1 | J9.1 63.5,43.94 61.98,42.42 52.88,42.42 J7.1 | R7.2 29.46,19.69 31.62,21.84 v31.62,24 | J7.1 50.75,42.37 48.64,40.26 48.64,28.09 47.37,26.82 47.37,24.51 v46.86,24
  Bottom 0.254: v46.86,24 v31.62,24
P27/RX2  (via drill 0.3 pad 0.64)
  Top 0.254: R7.1 v26.67,19.69
  Bottom 0.254: v26.67,19.69 26.67,18.67 26.92,18.42 U3.27
P28  (via drill 0.3 pad 0.64)
  Top 0.254: J9.2 64.26,52.7 65.02,51.94 65.02,43.18 62.23,40.39 52.85,40.39 J7.2 49.51,40.37 49.15,40 49.15,27.94 47.88,26.67 47.88,23.5 v47.5,23.11 | v30.35,23.11 30.23,23.11 R8.2
  Bottom 0.254: v47.5,23.11 v30.35,23.11
P28/TX2  (via drill 0.3 pad 0.64)
  Top 0.254: v26.67,20.96 26.67,21.08 R8.1
  Bottom 0.254: U3.28 v26.67,20.96
P29/CAN_TX2  (via drill 0.3 pad 0.64)
  Top 0.406: U2.1 22.86,20.7 TX.- v24.77,21.46
  Bottom 0.406: U3.29 25.4,23.5 24.77,22.86 v24.77,21.46
P30/CAN_RX2  (via drill 0.3 pad 0.64)
  Top 0.406: U2.4 19.05,21.08 RX.- 18.29,21.46 v17.78,20.96
  Bottom 0.406: U3.30 22.86,26.04 v17.78,20.96
RD+  (via drill 0.3 pad 0.64)
  Top 0.406: U4.11 v23.5,32.38 23.5,31.5 R44.2
  Bottom 0.254: U3.35 25.79,38.73 23.5,36.45 23.49,36.45 23.5,36.44 21.85,34.8 21.84,34.8 21.72,34.67 21.72,34.42 21.84,34.29 22.61,34.29 22.73,34.16 22.73,33.91 22.61,33.78 21.84,33.78 21.72,33.66 21.72,33.4 21.84,33.27 22.61,33.27 22.73,33.15 22.73,32.89 22.61,32.77 21.84,32.77 21.72,32.64 21.72,32.38 21.84,32.26 23.37,32.26 v23.5,32.38
RD-  (via drill 0.3 pad 0.64)
  Top 0.406: U4.9 v20.95,32.38 20.95,31.5 R45.1
  Bottom 0.254: v20.95,32.38 20.95,35.18 27.05,41.27 U3.36
RESET  (via drill 0.3 pad 0.64)
  Top 0.254: J6.1 v33.02,2.41
  Top 0.406: R32.1 14.86,7.24 v14.41,6.79 13.4,6.79 RST.- 6.1,6.73 RESET.P$2
  Bottom 0.254: U3.4 51.31,43.81
  Bottom 0.305: 51.31,43.81 54.48,43.81 59.94,38.35 59.94,29.59 J11.3
  Bottom 0.406: J11.3 63.5,10.67 53.98,1.14 33.27,1.14 | 33.27,1.14 33.02,1.14 | 33.02,1.14 32.77,1.14 | v33.02,2.41 33.02,1.14 | 32.77,1.14 33.02,1.4 33.27,1.14 | v14.41,6.79 14.41,5.92 19.19,1.14 32.77,1.14
RX+
  Top 0.254: J3.3 17.39,37.08 19.68,39.37 22.23,39.37 23.5,40.64 U4.6
RX-
  Top 0.254: J3.6 16.89,40.14 17.14,39.88 17.14,38.73 17.27,38.61 17.53,38.61 17.65,38.73 17.65,39.9 17.88,40.13 20.7,40.13 20.95,40.39 U4.8
TD+  (via drill 0.3 pad 0.64)
  Top 0.406: U4.16 v29.84,32.51 29.84,31.5 R42.2
  Bottom 0.254: v29.84,32.51 29.72,32.51 28.83,31.62 26.59,31.62 26.38,31.83 26.38,33.11 26.92,33.66 U3.33
TD-  (via drill 0.3 pad 0.64)
  Top 0.406: U4.14 v27.3,32.26 27.3,31.5 R43.1
  Bottom 0.254: v27.3,32.26 28.57,32.26 29.72,33.4 29.72,35.81 30.1,36.2 U3.34
TX+
  Top 0.254: J3.1 17.26,35.04 20.32,38.1 27.3,38.1 29.84,40.64 U4.1
TX-
  Top 0.254: J3.2 17.26,36.06 19.94,38.73 24.89,38.73 25.02,38.86 25.02,39.37 25.15,39.5 25.4,39.5 25.53,39.37 25.53,38.86 25.65,38.73 26.56,38.73 27.3,39.48 U4.3
USBD+
  Bottom 0.406: J5.DP 11.34,15.65 16.51,20.83 24.26,28.58 U3.31
USBD-
  Bottom 0.406: U3.32 24.8,31.12 15.24,21.56 J5.DM

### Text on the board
tPlace: TX2/P28 | RX2/P27 | GND | P7 | P6 | P5 | P21 | P22 | P9 | P10 | P23 | P24 | P25 | P26 | P8 | PWM | PWM | PWM | RX1 | RX2 | TX1 | TX2 | 5V | 5V | GND | GND | 5V | MISO | SCK | MOSI | RST | GND | ADC0 | RX3 | ADC1 | TX3 | 5V | 5V | GND | GND | CANL | CANH | RST | 3V3 | 5V | GND | GND | VIN | P15 | P16 | P17 | P18 | P19 | P20
bPlace: www.seeedstudio.com | by Seeed Studio | v0.9b 11/15/2012 | Mbed Shield
Milling: with copper | with copper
